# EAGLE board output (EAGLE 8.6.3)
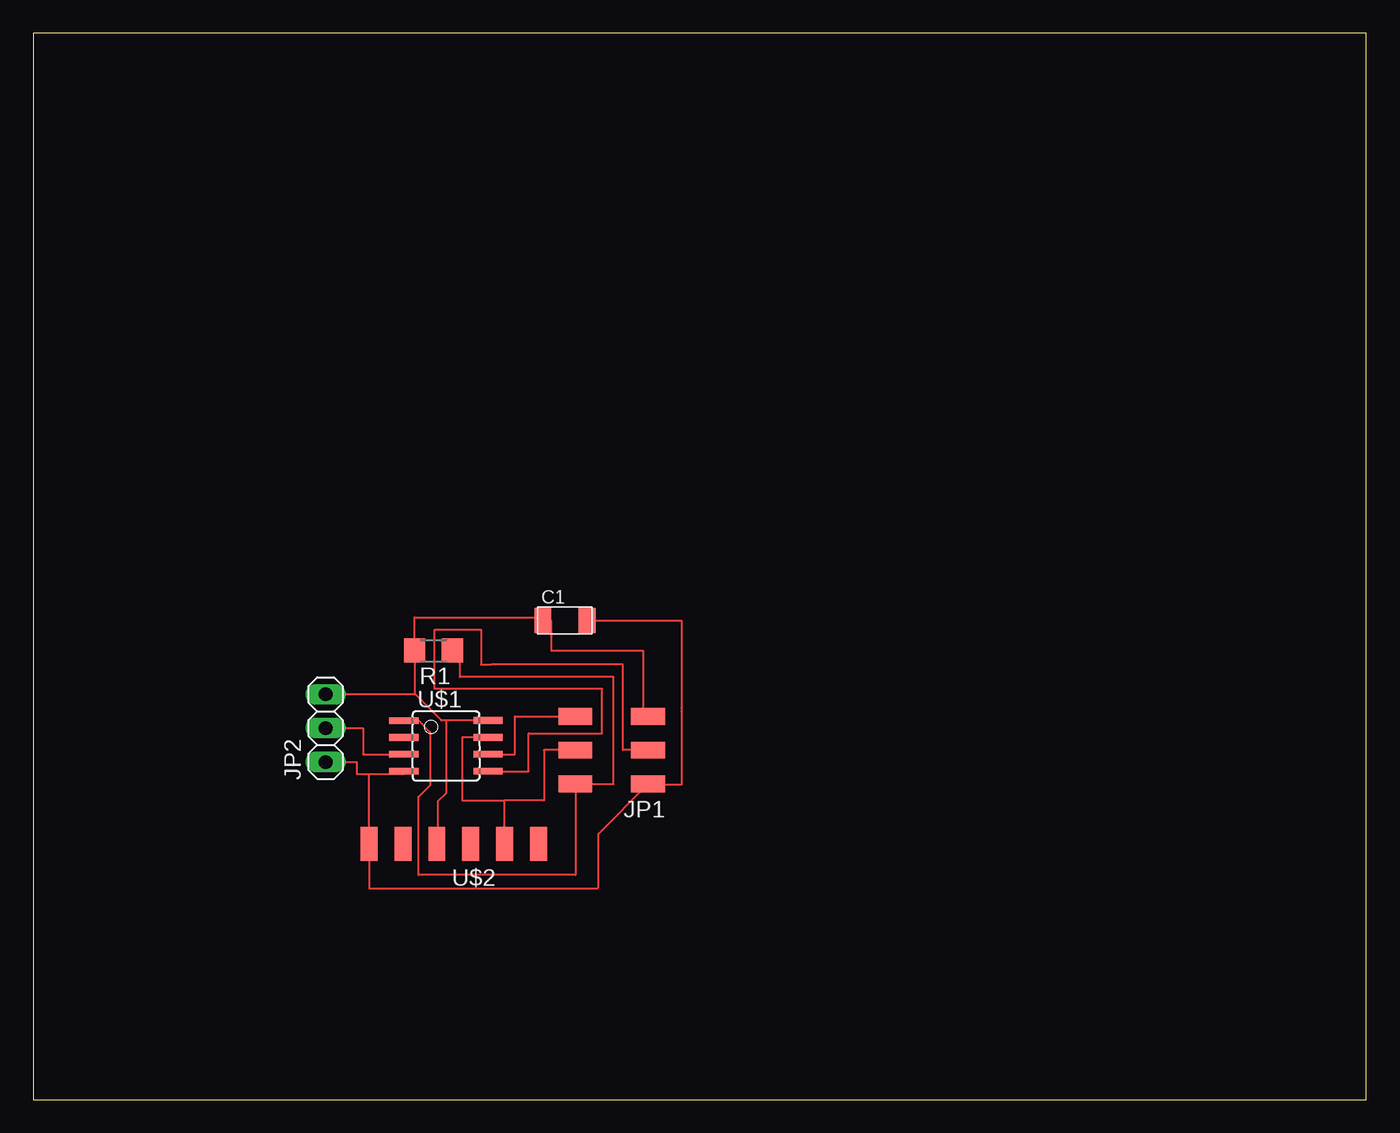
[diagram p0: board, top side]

Size 100 x 80 mm. Coordinates in mm from the lower left corner, seen from the top.
Outline: 0,0 100,0 100,80 0,80 0,0
Copper layers (1*16): Top 0.035mm / dielectric 1.5mm / Bottom 0.035mm
Design rules "default": minimum track width 6mil, minimum drill 0.35mm, track to track 6mil, track to pad 6mil, pad to pad 6mil, via to via 6mil, smd to smd 6mil, copper to edge 40mil, drill to drill 6mil, minimum pad ring 10mil, minimum via ring 8mil, stop-mask expansion 4mil, vias tented up to drill 0mil, thermal gap 10mil

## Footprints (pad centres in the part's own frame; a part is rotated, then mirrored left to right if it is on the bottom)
C1206FAB = smd 1.27 x 1.905: 1 -1.651,0; 2 1.651,0
2X03SMD = smd 2.54 x 1.27: 1 -2.54,2.54; 2 2.92,2.54; 3 -2.54,0; 4 2.92,0; 5 -2.54,-2.54; 6 2.92,-2.54
1X03 = drill 1.016 long: 1 -2.54,0; 2 0,0; 3 2.54,0
R1206 = smd 1.6 x 1.803: 1 -1.422,0; 2 1.422,0
SOIC8 = smd 0.5 x 2.2: 1 -1.905,-3.154; 2 -0.645,-3.154; 3 0.625,-3.154; 4 1.895,-3.154; 5 1.905,3.154; 6 0.635,3.154; 7 -0.635,3.154; 8 -1.905,3.154
1X06SMD = smd 2.54 x 1.27: 1 0,6.35; 2 0,3.81; 3 0,1.27; 4 0,-1.27; 5 0,-3.81; 6 0,-6.35

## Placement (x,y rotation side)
C1  [C1206FAB]  39.88,35.94 0 top
JP1  [2X03SMD]  43.59,26.21 180 top
JP2  [1X03]  21.93,27.86 90 top
R1  [R1206]  30.02,33.68 180 top
U$1  ATTINY45SI  [SOIC8]  30.96,26.53 270.1 top
U$2  FTDI-SMD-HEADER  [1X06SMD]  31.55,19.18 90 top

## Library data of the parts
C1 JP1 R1 U$1 U$2 = fab
JP2 = pinhead

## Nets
N$1: C1.1 JP1.5 JP2.3 R1.2 U$1.8 U$2.3
N$2: JP1.4 U$1.7 U$2.5
N$3: JP1.6 U$1.6
N$4: JP1.3 U$1.5
N$5: C1.2 JP1.1 JP2.1 U$1.4 U$2.1
N$6: JP2.2 U$1.3
N$7: JP1.2 R1.1 U$1.1

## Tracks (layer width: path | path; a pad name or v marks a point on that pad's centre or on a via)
N$1
  Top 0.152: 28.6,30.45 28.6,30.4 | 28.6,30.4 JP2.3 | 28.6,30.45 R1.2 28.6,36.17 38.23,36.17 C1.1 38.85,35.94 38.85,33.69 45.76,33.69 45.76,28.8 46.13,28.8 | 28.6,30.4 28.6,30.39 | U$1.8 30.96,28.44 | U$2.3 30.34,19.18 30.34,22.35 30.96,22.97 30.96,28.44 | 30.96,28.44 30.61,28.44 28.6,30.45 | 46.13,29.2 46.13,28.8 | 46.13,28.8 JP1.5
N$2
  Top 0.152: U$1.7 32.17,27.17 32.17,22.44 35.36,22.44 | U$2.5 35.36,22.44 | 35.36,22.44 38.3,22.44 38.3,26.21 JP1.4
N$3
  Top 0.152: U$1.6 36.13,25.9 36.13,28.75 JP1.6
N$4
  Top 0.152: U$1.5 37.16,24.63 37.16,27.47 42.69,27.47 42.69,30.81 30.11,30.81 30.11,35.26 33.59,35.26 33.59,32.63 34.37,32.63 34.68,32.63 44.23,32.63 44.23,26.21 JP1.3
N$5
  Top 0.152: JP2.1 24.26,25.32 24.26,24.42 25.2,24.42 | 25.2,24.42 27.81,24.42 U$1.4 | 25.2,24.42 U$2.1 25.2,15.84 42.33,15.84 42.39,15.9 42.39,19.94 JP1.1 46.19,23.61 48.63,23.61 48.63,29.11 48.63,29.36 48.63,35.94 C1.2
N$6
  Top 0.152: JP2.2 24.73,27.86 24.73,25.9 U$1.3
N$7
  Top 0.152: U$1.1 28.9,28.43 29.77,27.56 29.77,23.58 28.91,22.72 28.91,16.85 40.67,16.85 JP1.2 43.54,23.67 43.54,31.7 32.02,31.7 32.02,33.68 R1.1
